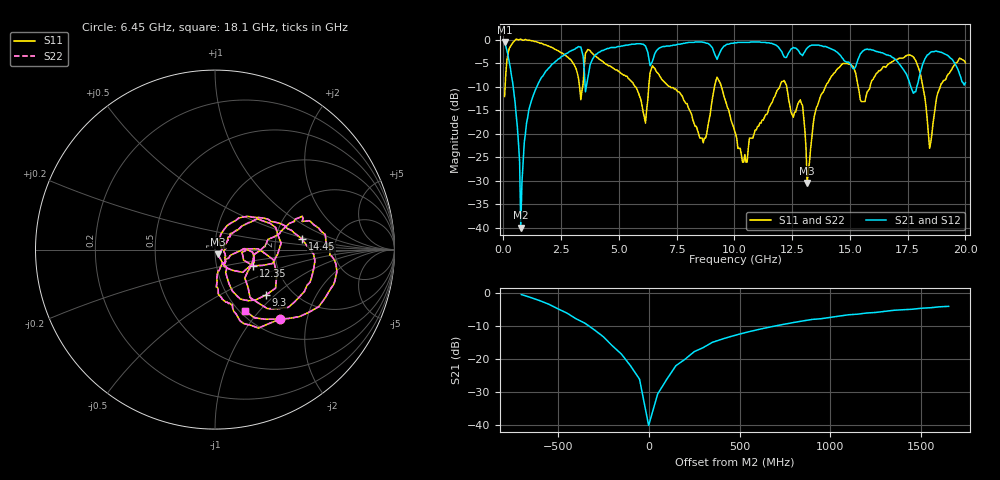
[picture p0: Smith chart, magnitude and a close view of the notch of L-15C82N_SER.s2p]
# MHZ S MA R 50
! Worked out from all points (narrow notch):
!   400 points, 50 MHz to 20 GHz, reference 50 ohm
!   highest |S21| = -0.45 dB at 50 MHz (marker M1); lowest = -40.0 dB at 750 MHz (marker M2)
!   notch at M2: 37.6 dB deep, 280 MHz wide at half that depth
!   lowest |S11| = -30.5 dB at 13.15 GHz (marker M3), VSWR 1.06, Z = 51.5 - j2.64 ohm
!   |S11| at or under -10 dB: 7.219 GHz to 9.137 GHz (1.918 GHz wide, 23.5 % of centre); 9.439 GHz to 11.96 GHz (2.522 GHz wide, 23.6 % of centre); 12.26 GHz to 13.94 GHz (1.678 GHz wide, 12.8 % of centre)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
!   |S22| runs from -30.5 to 0.2 dB; largest |S21 - S12| = 0
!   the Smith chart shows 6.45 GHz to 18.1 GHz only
!   S11 on the Smith chart (normalised r, x): 6.45 GHz: 1.29, -1.39; 9.3 GHz: 1.48, -0.88; 12.35 GHz: 1.50, -0.29; 14.45 GHz: 2.85, +0.43; 18.1 GHz: 1.05, -0.84
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50  0.25 71.9  0.95 -12.8  0.95 -12.8  0.25 71.9
600  1.01 10.6  0.12 -81.3  0.12 -81.3  1.01 10.6
750  1.02 4.7  0.01 -71.2  0.01 -71.2  1.02 4.7
900  1 -1.4  0.08 79.6  0.08 79.6  1 -1.4
1250  0.98 -12.1  0.24 72.1  0.24 72.1  0.98 -12.1
3400  0.29 -25.1  0.75 -7.0  0.75 -7.0  0.29 -25.1
4000  0.67 -57.5  0.7 33.1  0.7 33.1  0.67 -57.5
6150  0.13 -51.7  0.86 -10.4  0.86 -10.4  0.13 -51.7
6450  0.53 -47.0  0.59 11.3  0.59 11.3  0.53 -47.0
6700  0.44 -69.0  0.8 9.1  0.8 9.1  0.44 -69.0
8650  0.08 -41.6  0.94 -16.6  0.94 -16.6  0.08 -41.6
9300  0.38 -41.8  0.67 -11.1  0.67 -11.1  0.38 -41.8
10050  0.1 -58.4  0.93 -16.7  0.93 -16.7  0.1 -58.4
12350  0.23 -23.1  0.73 -27.8  0.73 -27.8  0.23 -23.1
12950  0.2 -39.3  0.68 -32.9  0.68 -32.9  0.2 -39.3
13150  0.03 -58.7  0.82 -29.5  0.82 -29.5  0.03 -58.7
13350  0.09 69.2  0.88 -35.6  0.88 -35.6  0.09 69.2
14450  0.49 6.7  0.74 -56.7  0.74 -56.7  0.49 6.7
16700  0.56 15.4  0.68 -60.9  0.68 -60.9  0.56 15.4
18100  0.38 -64.0  0.5 -16.3  0.5 -16.3  0.38 -64.0
18450  0.07 -42.6  0.72 -33.1  0.72 -33.1  0.07 -42.6
20000  0.57 -44.4  0.35 -48.5  0.35 -48.5  0.57 -44.4
